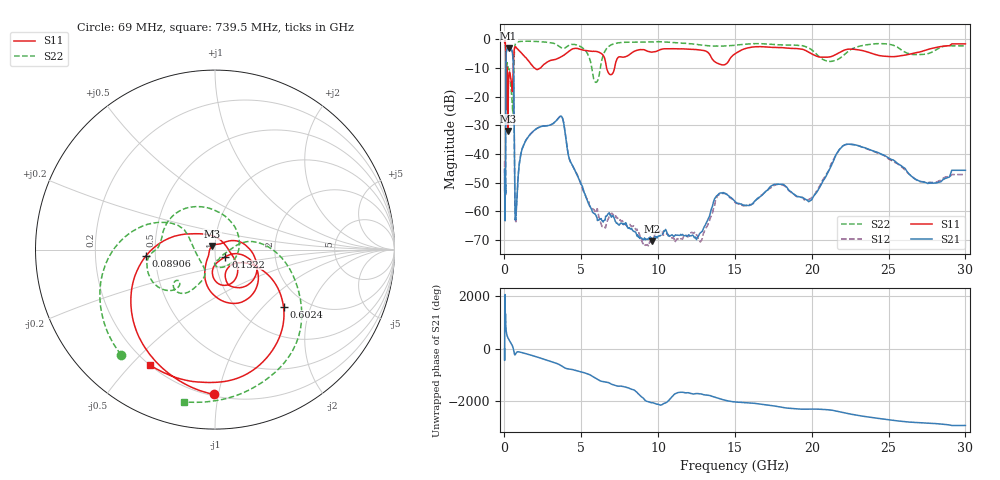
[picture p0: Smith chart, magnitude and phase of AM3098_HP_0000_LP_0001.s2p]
! Date/Time: Thu, Feb 28, 2019 8:30 AM
! Network Analyzer: Agilent Technologies E8364B Rev: A.07.50.67
! Sweep from 0.010 to 30.000 GHz, 1601 Points, Sweep Type: LOG
! Power Supply: 5.022 V, 0.002 A
# Hz S DB R 50
!freq MagS11 AngS11 MagS21 AngS21 MagS12 AngS12 MagS22 AngS22
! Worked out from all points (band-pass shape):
!   1601 points, 10 MHz to 30 GHz, reference 50 ohm
!   highest |S21| = -2.98 dB at 265.1 MHz (marker M1); lowest = -70.3 dB at 9.634 GHz (marker M2)
!   |S21| within 3 dB of the highest: 103.7 MHz to 546 MHz (442.3 MHz wide, 136 % of centre)
!   lowest |S11| = -31.9 dB at 227 MHz (marker M3), VSWR 1.05, Z = 48.4 + j1.96 ohm
!   |S11| at or under -10 dB: 175.4 MHz to 571 MHz (395.6 MHz wide, 106 % of centre); 1.965 GHz to 2.327 GHz (361.5 MHz wide, 16.8 % of centre); 6.651 GHz to 7.164 GHz (513.2 MHz wide, 7.43 % of centre)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
!   |S22| runs from -25.9 to -0.5 dB; largest |S21 - S12| = 0.01
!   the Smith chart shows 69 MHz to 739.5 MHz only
!   S11 on the Smith chart (normalised r, x): 69 MHz: 0.21, -0.97; 89.06 MHz: 0.44, -0.04; 132.2 MHz: 1.12, -0.09; 602.4 MHz: 1.55, -1.32; 739.5 MHz: 0.20, -0.57
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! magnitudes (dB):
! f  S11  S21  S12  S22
! 10 MHz  -0.4  -45.2  -42.6  -0.5
! 38.04 MHz  -0.5  -61.2  -61.2  -0.8
! 69 MHz  -1.9  -51.0  -53.9  -2.1
! 89.06 MHz  -8.2  -18.2  -18.2  -10.0
! 132.2 MHz  -23.1  -3.8  -3.7  -11.5
! 144.7 MHz  -13.2  -3.5  -3.5  -10.1
! 187.7 MHz  -11.7  -3.4  -3.4  -8.3
! 227 MHz  -31.9  -3.1  -3.0  -9.9
! 265.1 MHz  -15.1  -3.0  -2.9  -10.4
! 550.5 MHz  -13.5  -6.3  -6.2  -25.9
! 602.4 MHz  -6.0  -14.4  -14.4  -12.3
! 679.2 MHz  -2.6  -57.9  -57.8  -2.2
! 739.5 MHz  -2.6  -61.5  -63.6  -1.2
! 1.044 GHz  -4.4  -40.7  -40.7  -0.7
! 2.084 GHz  -10.5  -31.2  -31.1  -0.7
! 3.704 GHz  -6.0  -26.8  -26.9  -2.9
! 5.959 GHz  -4.2  -61.4  -60.5  -15.0
! 7.926 GHz  -5.9  -64.1  -64.8  -1.0
! 9.634 GHz  -4.4  -70.3  -69.9  -0.9
! 19.7 GHz  -4.2  -56.1  -56.0  -2.7
! 22.56 GHz  -3.4  -36.6  -36.6  -3.5
! 30 GHz  -1.6  -45.6  -47.1  -2.2
